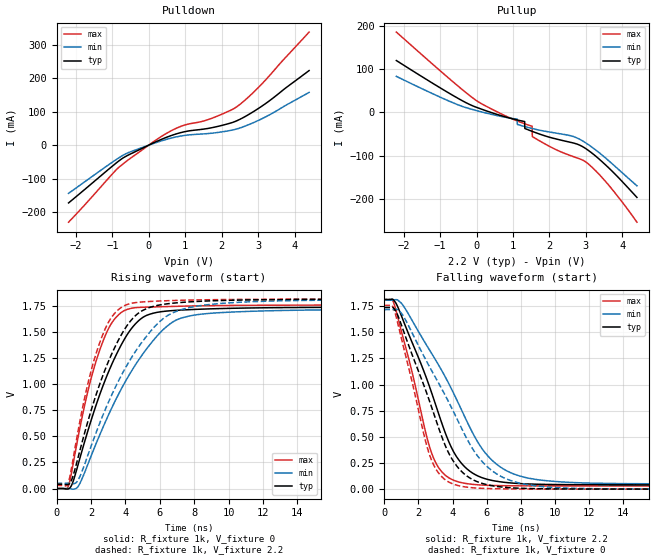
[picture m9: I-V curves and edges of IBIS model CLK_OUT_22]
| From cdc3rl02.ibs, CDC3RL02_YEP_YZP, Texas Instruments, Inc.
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[Model]   CLK_OUT_22
Model_type  Output
Vref =   1.8
Rref =   1M
Cref =   30p
Vmeas =   0.9
| variable   typ   min   max
C_comp   37.25pF   14.85pF   49.61pF
| C_pullup   31.26pF   14.85pF   36.90pF
| C_pulldown   43.24pF   39.36pF   49.61pF
[Temperature Range]   40   100   -40
| Ambient temperature   25   85   -40
[Voltage range]   2.2   2   2.4
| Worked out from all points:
|   slope of the pulldown table from 0 to 0.33 V, typ, clamps not added: 20 ohm
|   slope of the pullup table from 0 to 0.33 V, typ, clamps not added: 33.5 ohm
|   rising waveform, R_fixture 1k, V_fixture 0: 20-80 % time 2.35ns typ, 3.32ns min, 1.6ns max; typ from 0 V to 1.74 V
|   falling waveform, R_fixture 1k, V_fixture 2.2: 20-80 % time 2.46ns typ, 3.49ns min, 1.6ns max; typ from 1.81 V to 0.041 V
|   rising waveform, R_fixture 1k, V_fixture 2.2: 20-80 % time 2.32ns typ, 3.23ns min, 1.58ns max; typ from 0.041 V to 1.81 V
|   falling waveform, R_fixture 1k, V_fixture 0: 20-80 % time 2.37ns typ, 3.35ns min, 1.55ns max; typ from 1.74 V to 0 V
[Pulldown]
| CLK_OUT_22
|   Voltage   I(typ)   I(min)   I(max)
-2.2V     -172.5mA   -144mA     -230mA
-855mV    -50.09mA   -40.31mA   -69.67mA
-565mV    -29.86mA   -22.59mA   -44.12mA
175mV     9.028mA    6.683mA    13.59mA
510mV     24.38mA    17.94mA    36.61mA
810mV     35.35mA    25.78mA    52.96mA
1.025V    41.03mA    29.59mA    61.3mA
1.735V    52.14mA    35.73mA    80.37mA
2.28V     67.13mA    44.76mA    105.9mA
2.5V      77.08mA    51.19mA    121.5mA
3.1V      116.1mA    78.65mA    182.4mA
4.4V      222.7mA    157.6mA    337.5mA
[Pullup]
| CLK_OUT_22
|   Voltage   I(typ)   I(min)   I(max)
-2.2V     119.5mA    83.1mA     184.9mA
-5mV      11.99mA    4.485mA    27.47mA
1.115V    -17.13mA   -15.34mA   -19.42mA
1.12V     -17.23mA   -27.44mA   -19.58mA
1.32V     -20.86mA   -32.29mA   -25.93mA
1.325V    -36.77mA   -32.4mA    -26.08mA
1.525V    -43.35mA   -36.82mA   -31.67mA
1.53V     -43.51mA   -36.93mA   -55.31mA
2.76V     -72.73mA   -58.7mA    -104.5mA
3.02V     -84.36mA   -71.18mA   -115.2mA
3.37V     -107.6mA   -92.83mA   -142.8mA
4.4V      -195.2mA   -168.5mA   -252.2mA
[Ramp]
| CLK_OUT_22
| variable   typ   min   max
dV/dt_r   1.05/2.36E-09   1.03/3.33E-09   1.06/1.60E-09
dV/dt_f   1.07/2.46E-09   1.06/3.50E-09   1.07/1.60E-09
R_load = 1k
[Rising Waveform]
| CLK_OUT_22
R_fixture =   1k
C_fixture =   0
L_fixture =   0
V_fixture =   0
V_fixture_min = 0
V_fixture_max = 0
|   Time   V(typ)   V(min)   V(max)
0s        9.559nV    28.61nV    2.329nV
709ps     -2.001mV   -228.5uV   32.89mV
1.301ns   256.5mV    31.82mV    530.8mV
2.029ns   662mV      319.1mV    1.065V
2.797ns   1.025V     622.4mV    1.45V
4.221ns   1.501V     1.087V     1.721V
5.109ns   1.648V     1.309V     1.736V
6.397ns   1.699V     1.55V      1.742V
8.413ns   1.717V     1.67V      1.749V
37.7ns    1.737V     1.717V     1.757V
[Falling Waveform]
| CLK_OUT_22
R_fixture =   1k
C_fixture =   0
L_fixture =   0
V_fixture =   2.2
V_fixture_min = 2
V_fixture_max = 2.4
|   Time   V(typ)   V(min)   V(max)
0s        1.814V     1.809V     1.814V
621ps     1.793V     1.811V     1.747V
1.157ns   1.593V     1.743V     1.413V
2.853ns   883mV      1.276V     310.5mV
3.413ns   610.5mV    1.121V     158.3mV
4.357ns   281.5mV    816.1mV    69mV
5.429ns   130.5mV    463.9mV    42.46mV
6.293ns   84.24mV    279.9mV    35.6mV
8.949ns   47.21mV    91.34mV    31.06mV
37.7ns    40.8mV     49.79mV    29.68mV
[Rising Waveform]
| CLK_OUT_22
R_fixture =   1k
C_fixture =   0
L_fixture =   0
V_fixture =   2.2
V_fixture_min = 2
V_fixture_max = 2.4
|   Time   V(typ)   V(min)   V(max)
0s        40.81mV    49.8mV     29.68mV
709ps     40.98mV    49.55mV    69.2mV
1.277ns   312.5mV    87.76mV    573.1mV
1.925ns   700.1mV    366.8mV    1.073V
2.653ns   1.064V     683.8mV    1.459V
3.341ns   1.336V     942.6mV    1.67V
4.237ns   1.591V     1.22V      1.769V
6.325ns   1.766V     1.642V     1.798V
8.893ns   1.796V     1.762V     1.808V
37.7ns    1.813V     1.809V     1.814V
[Falling Waveform]
| CLK_OUT_22
R_fixture =   1k
C_fixture =   0
L_fixture =   0
V_fixture =   0
V_fixture_min = 0
V_fixture_max = 0
|   Time   V(typ)   V(min)   V(max)
0s        1.737V     1.717V     1.757V
621ps     1.716V     1.719V     1.692V
1.085ns   1.531V     1.663V     1.385V
2.765ns   787.2mV    1.136V     278.6mV
3.621ns   398.5mV    881.1mV    84.19mV
4.269ns   216.7mV    669.2mV    36.83mV
5.237ns   86.77mV    370.5mV    12.54mV
6.149ns   38.33mV    198mV      5.491mV
8.861ns   4.93mV     31.87mV    1.323mV
37.7ns    -9.786uV   -13.07uV   -6.671uV
